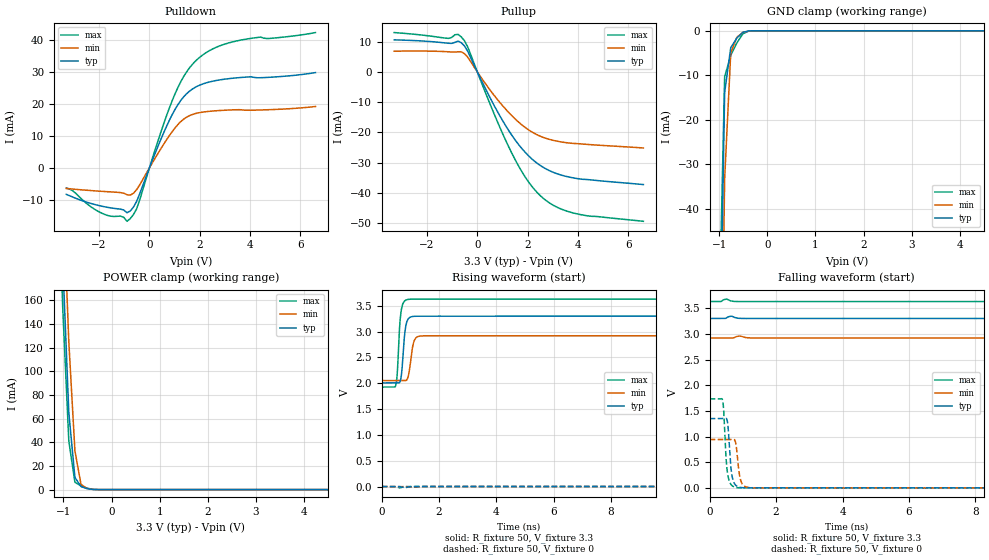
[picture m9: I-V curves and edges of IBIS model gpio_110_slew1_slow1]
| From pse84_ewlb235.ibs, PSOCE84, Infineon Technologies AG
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[Model] gpio_110_slew1_slow1
Model_type I/O
Enable   Active-High
Vinl  =  0.99
Vinh  =  2.31
Vmeas =  1.65
Cref  =  15e-12
| Capacitance   typ   min   max
C_comp   1.09946e-12   1.08623e-12   1.11440e-12
| Variables   typ   min   max
[GND Clamp Reference]   0   0   0
[POWER Clamp Reference]   3.3   2.92   3.63
[Pulldown Reference]   0   0   0
[Pullup Reference]   3.3   2.92   3.63
[Temperature Range]   25   125   -40
[Voltage Range]   3.3   2.92   3.63
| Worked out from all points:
|   slope of the pulldown table from 0 to 0.495 V, typ, clamps not added: 51.4 ohm
|   slope of the pullup table from 0 to 0.495 V, typ, clamps not added: 59.6 ohm
|   GND clamp passes 1 mA (typ) near -0.57 V on its own axis
|   POWER clamp passes 1 mA (typ) near -0.52 V on its own axis
|   falling waveform, R_fixture 50, V_fixture 3.3: 20-80 % time 654ns typ, 981ns min, 355ns max; typ from 3.3 V to 2.01 V
|   falling waveform, R_fixture 50, V_fixture 0: 20-80 % time 96.9ps typ, 106ps min, 92.4ps max; typ from 1.35 V to 0 V
|   rising waveform, R_fixture 50, V_fixture 3.3: 20-80 % time 114ps typ, 134ps min, 102ps max; typ from 2.01 V to 3.3 V
|   rising waveform, R_fixture 50, V_fixture 0: 20-80 % time 659ns typ, 959ns min, 406ns max; typ from 0 V to 1.34 V
[GND Clamp]
| Voltage   I(typ)   I(min)   I(max)
-1.65V    -892.5mA   -911.9mA   -883.9mA
-1.015V   -92.32mA   -129.7mA   -71.28mA
-888.3mV  -13.83mA   -33.21mA   -10.31mA
-761.4mV  -3.792mA   -4.944mA   -5.509mA
-634.5mV  -1.622mA   -1.436mA   -2.707mA
-507.6mV  -326.2uA   -352.3uA   -651.6uA
-380.7mV  -13.48uA   -32.14uA   -19.55uA
-253.8mV  -189.4nA   -1.276uA   -466.7nA
6.6V      0A         0A         0A
[POWER Clamp]
| Voltage   I(typ)   I(min)   I(max)
-1.523V   838.1mA    872.9mA    823.9mA
-1.142V   346.5mA    405.1mA    310.5mA
-1.015V   193mA      257.4mA    153.9mA
-888.3mV  64.97mA    124.9mA    40.96mA
-761.4mV  10.28mA    32.7mA     6.184mA
-634.5mV  2.553mA    4.346mA    3.067mA
-507.6mV  805.9uA    960.7uA    1.159mA
-253.8mV  1.454uA    10.02uA    1.678uA
6.6V      0A         0A         0A
[Pulldown]
| Voltage   I(typ)   I(min)   I(max)
-3.3V     -8.212mA   -6.385mA   -6.208mA
-2.03V    -11.66mA   -7.198mA   -13.53mA
-1.142V   -12.83mA   -7.669mA   -15.01mA
-888.3mV  -13.95mA   -8.319mA   -16.62mA
-507.6mV  -10.46mA   -6.799mA   -12.77mA
455.2mV   8.891mA    5.988mA    11.13mA
1.024V    18.33mA    12.54mA    23.2mA
1.366V    22.23mA    15.26mA    28.56mA
1.821V    25.16mA    16.97mA    33.26mA
2.503V    27.06mA    17.77mA    37.09mA
3.3V      28mA       18.13mA    39.33mA
6.6V      29.77mA    19.2mA     42.25mA
[Pullup]
| Voltage   I(typ)   I(min)   I(max)
-3.3V     10.56mA    6.824mA    12.97mA
-1.142V   9.434mA    6.617mA    11.05mA
-761.4mV  10.16mA    6.619mA    12.36mA
-634.5mV  9.61mA     6.607mA    11.54mA
-380.7mV  6.811mA    4.857mA    8.263mA
682.8mV   -11.29mA   -7.892mA   -14.14mA
1.479V    -22.19mA   -15.35mA   -28.59mA
2.048V    -27.81mA   -19.21mA   -36.47mA
2.731V    -32.06mA   -21.96mA   -42.48mA
3.3V      -34mA      -23.09mA   -45.19mA
4.051V    -35.35mA   -23.76mA   -47.06mA
6.6V      -37.22mA   -25.13mA   -49.35mA
[Ramp]
dV/dt_r   0.806899/0.659323u  0.556932/0.95876u  1.03904/0.406228u
dV/dt_f   0.774754/0.653549u  0.514858/0.981159u  1.02149/0.35469u
R_load = 50
[Falling Waveform]
R_fixture = 50
V_fixture = 3.3
V_fixture_min = 2.92
V_fixture_max = 3.63
| Time   V(typ)   V(min)   V(max)
0s        3.3V       2.92V      3.63V
506.9ps   3.312V     2.92V      3.677V
123.5ns   3.3V       2.92V      3.587V
289.2ns   3.181V     2.917V     2.871V
452.1ns   2.866V     2.849V     2.416V
615ns     2.609V     2.716V     2.198V
818.6ns   2.395V     2.555V     2.072V
1.221us   2.184V     2.338V     1.975V
1.854us   2.067V     2.176V     1.937V
4us       2.009V     2.062V     1.928V
[Falling Waveform]
R_fixture = 50
V_fixture = 0
V_fixture_min = 0
V_fixture_max = 0
| Time   V(typ)   V(min)   V(max)
0s        1.349V     941.3mV    1.732V
388.4ps   1.349V     941.1mV    1.709V
425.3ps   1.349V     941.2mV    1.478V
514.8ps   1.339V     941.3mV    409.5mV
636.4ps   413.3mV    941.3mV    70.21mV
690.4ps   181.6mV    942.5mV    34.31mV
785.6ps   49.61mV    870.1mV    8.847mV
895ps     11.88mV    262.1mV    968.7uV
980.3ps   3.481mV    77.25mV    586uV
4us       17.3nV     488.5nV    8.402nV
[Rising Waveform]
R_fixture = 50
V_fixture = 3.3
V_fixture_min = 2.92
V_fixture_max = 3.63
| Time   V(typ)   V(min)   V(max)
0s        2.007V     2.052V     1.927V
485.3ps   2.007V     2.052V     1.952V
539.5ps   2.007V     2.052V     2.174V
619.5ps   2.013V     2.052V     3.054V
686.7ps   2.163V     2.052V     3.432V
836.2ps   3.098V     2.053V     3.61V
1.03ns    3.288V     2.528V     3.629V
1.207ns   3.299V     2.887V     3.629V
1.833ns   3.299V     2.92V      3.629V
4us       3.3V       2.92V      3.63V
[Rising Waveform]
R_fixture = 50
V_fixture = 0
V_fixture_min = 0
V_fixture_max = 0
| Time   V(typ)   V(min)   V(max)
0s        14.93nV    475.9nV    8.654nV
131.5ns   450.1uV    120.7uV    58.01mV
262.1ns   82.38mV    5.128mV    514.4mV
380.8ns   275.7mV    44.59mV    918.6mV
503ns     492.4mV    124.5mV    1.209V
665.9ns   742.1mV    255.1mV    1.427V
869.5ns   962.2mV    414.1mV    1.559V
1.272us   1.173V     647.9mV    1.666V
1.872us   1.281V     814.2mV    1.713V
4us       1.345V     928.2mV    1.732V
